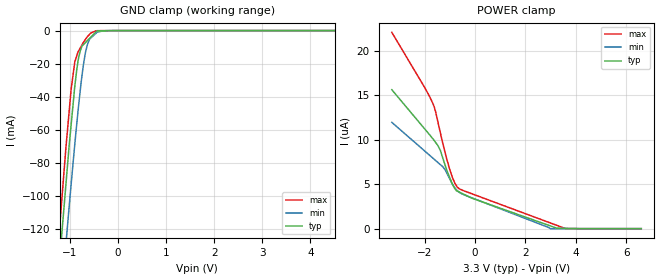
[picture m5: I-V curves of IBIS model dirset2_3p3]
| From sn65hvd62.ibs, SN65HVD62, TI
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|   dirset2_3p3 Model
[Model]   dirset2_3p3
Model_type   Input
Vinl = 0.99
Vinh = 2.3
|   typ   min   max
|   (nom PVT)   (fast PVT)   (slow PVT)
 C_comp   1.384e-12   1.365e-12   1.424e-12
| Where nom  PVT is Nominal Process, 3.3V, 27C
|   Fast PVT is Strong Process,  3.6V, -40C
|   Slow PVT is Weak Process,   3V, 125C
[Voltage Range]   3.3   3   3.6
|Ambient Temperature   25   85   -40
|Junction Temperature
[Temperature Range]   27   125   -40
[Power Clamp Reference]   3.3   3   3.6
[GND Clamp Reference]   0   0   0
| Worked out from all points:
|   GND clamp passes 1 mA (typ) near -0.46 V on its own axis
[GND Clamp]
|   Voltage   I(typ)   I(min)   I(max)
-3.3V     -966.6mA   -966.7mA   -974.3mA
-1.215V   -140.7mA   -176mA     -120.6mA
-1.178V   -127.2mA   -163.2mA   -107mA
-1.08V    -93.06mA   -129.2mA   -70.77mA
-1.038V   -78.42mA   -115mA     -57.1mA
-972mV    -57.11mA   -93.09mA   -35.62mA
-896.4mV  -33.94mA   -68.98mA   -19.07mA
-818.4mV  -16.79mA   -45.91mA   -12.42mA
-669mV    -7.093mA   -12.57mA   -5.071mA
-585mV    -4.624mA   -5.046mA   -2.167mA
-453.6mV  -760.2uA   -1.583mA   -110.1uA
6.6V      0A         0A         0A
[POWER Clamp]
|   Voltage   I(typ)   I(min)   I(max)
-3.3V     15.61uA    11.94uA    22.04uA
-2.045V   11.37uA    8.845uA    16.09uA
-1.667V   10.08uA    7.914uA    14.04uA
-1.562V   9.684uA    7.657uA    13.14uA
-1.376V   8.803uA    7.198uA    10.8uA
-1.179V   7.081uA    6.596uA    8.471uA
-1.015V   5.83uA     5.67uA     6.777uA
-799.2mV  4.504uA    4.578uA    5.11uA
-622.8mV  4.109uA    4.085uA    4.474uA
2.997V    303.1nA    0A         634.4nA
3.596V    39.85nA    0A         0A
6.6V      0A         0A         0A
